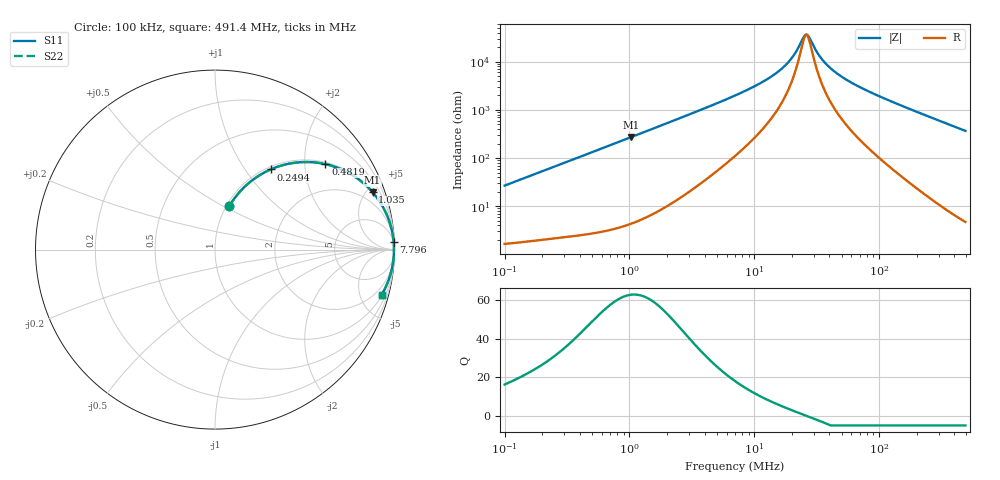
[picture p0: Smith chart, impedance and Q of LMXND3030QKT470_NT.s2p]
! LMXND3030QKT470_NT  S-PARAMETER MODEL  ( Standard Model )
! Model Generated by TAIYO YUDEN Corporation (https://www.yuden.co.jp/en/)
! Version 1.0
! TAIYO YUDEN Control No. 20250724
! Copyright(c) 2025 TAIYO YUDEN CO.,LTD. All Rights Reserved.
! Product Description (link to TY-COMPAS)
! https://ds.yuden.co.jp/TYCOMPAS/or/detail?pn=LMXND3030QKT470MNT&u=M
! Products Name : Inductors
! Characteristics :
!  Inductance : 47 [uH] , SRF(min) : 17 [MHz] , DC Resistance(max) : 1.32 [Ohm]
!  Rated Current : Saturation  325 [m A] , Temp Rise  470 [m A] (40 [degC])
!  Case Size : 3.0 x 3.0 / 0.118 x 0.118 [mm/inch] , Thickness : 1.5 / 0.059 [mm/inch]
!  (Conditions: Temperature = 25 [degC] , DC Bias Current = 0 [A])
! External Node Assignments :
!  1  o---GGG---o  2
! GND o---------o GND
! Frequency Range : 0.1MHz  -  491.415554MHz  [ 402 STEP ]
# MHz S RI R 50
! Freq[MHz].  S11 Real  S11 Imag  S21 Real  S21 Imag  S12 Real  S12 Imag  S22 Real  S22 Imag
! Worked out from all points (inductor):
!   401 points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, 100 kHz to 491.4 MHz, reference 50 ohm
!   read as one part in series: L = 42.4 uH near 104.3 kHz
!   highest Q = 62.7 at 1.035 MHz (marker M1), where L = 41.9 uH
!   self-resonance near 25.63 MHz
!   S11 on the Smith chart (normalised r, x): 100 kHz: 1.03, +0.53; 249.4 kHz: 1.04, +1.32; 481.9 kHz: 1.05, +2.54; 1.035 MHz: 1.09, +5.46; 7.796 MHz: 4, +45; 491.4 MHz: 1.09, -7.33
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0.1  0.0799 0.242  0.9201 -0.242  0.9201 -0.242  0.0799 0.242
0.159599  0.1636 0.3485  0.8364 -0.3485  0.8364 -0.3485  0.1636 0.3485
0.249362  0.3094 0.4463  0.6906 -0.4463  0.6906 -0.4463  0.3094 0.4463
0.415258  0.5445 0.4866  0.4555 -0.4866  0.4555 -0.4866  0.5445 0.4866
0.481857  0.6151 0.4762  0.3849 -0.4762  0.3849 -0.4762  0.6151 0.4762
0.706372  0.772 0.411  0.228 -0.411  0.228 -0.411  0.772 0.411
1.035496  0.8777 0.3198  0.1223 -0.3198  0.1223 -0.3198  0.8777 0.3198
1.72439  0.9507 0.2079  0.0493 -0.2079  0.0493 -0.2079  0.9507 0.2079
7.010104  0.9947 0.05  0.0053 -0.05  0.0053 -0.05  0.9947 0.05
7.795923  0.9953 0.0441  0.00473 -0.0441  0.00473 -0.0441  0.9953 0.0441
12.1806  0.9967 0.0243  0.00334 -0.0243  0.00334 -0.0243  0.9967 0.0243
16.75321  0.9971 0.0133  0.00291 -0.0133  0.00291 -0.0133  0.9971 0.0133
20.28409  0.9972 0.00744  0.00278 -0.00744  0.00278 -0.00744  0.9972 0.00744
25.62539  0.9973 0.000596  0.00272 -0.000596  0.00272 -0.000596  0.9973 0.000596
27.31217  0.9973 -0.00125  0.00271 0.00125  0.00271 0.00125  0.9973 -0.00125
29.11  0.9973 -0.0031  0.00272 0.0031  0.00272 0.0031  0.9973 -0.0031
35.24518  0.9972 -0.00876  0.00278 0.00876  0.00278 0.00876  0.9972 -0.00876
45.48238  0.997 -0.0168  0.00299 0.0168  0.00299 0.0168  0.997 -0.0168
66.67429  0.9963 -0.0312  0.00368 0.0312  0.00368 0.0312  0.9963 -0.0312
120.8815  0.9932 -0.0635  0.00679 0.0635  0.00679 0.0635  0.9932 -0.0635
248.962  0.9788 -0.1338  0.0212 0.1338  0.0212 0.1338  0.9788 -0.1338
491.4156  0.9279 -0.2523  0.0721 0.2523  0.0721 0.2523  0.9279 -0.2523
